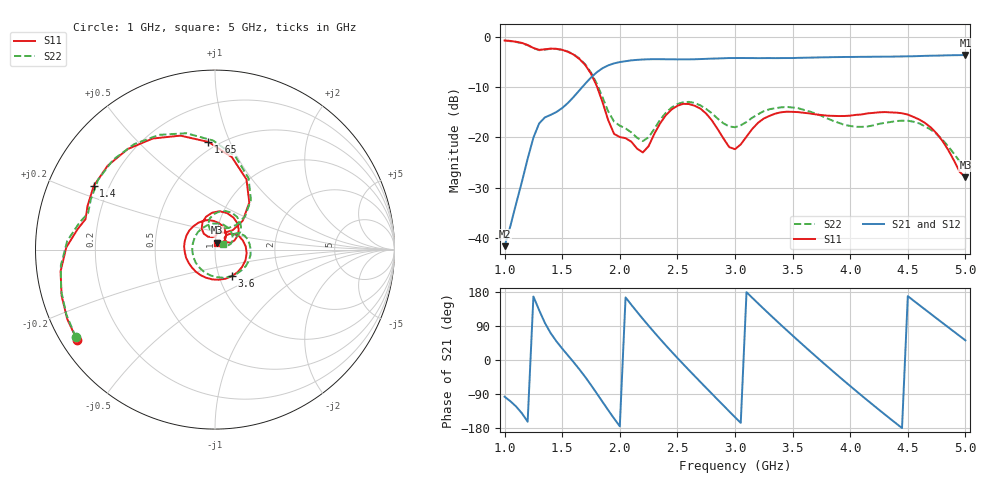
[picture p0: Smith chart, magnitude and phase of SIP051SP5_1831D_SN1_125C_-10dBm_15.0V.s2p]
# GHz  S  dB  R  50
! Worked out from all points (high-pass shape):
!   81 points, 1 GHz to 5 GHz, reference 50 ohm
!   highest |S21| = -3.63 dB at 5 GHz (marker M1); lowest = -41.6 dB at 1 GHz (marker M2)
!   |S21| within 3 dB of the highest: 1.827 GHz to end of sweep
!   lowest |S11| = -27.9 dB at 5 GHz (marker M3), VSWR 1.08, Z = 51.1 + j3.89 ohm
!   |S11| at or under -10 dB: 1.803 GHz to end of sweep
!   |S22| runs from -25.3 to -0.8 dB; largest |S21 - S12| = 0.0015
!   S11 on the Smith chart (normalised r, x): 1 GHz: 0.05, -0.30; 1.4 GHz: 0.14, +0.24; 1.65 GHz: 0.45, +0.84; 3.6 GHz: 1.15, -0.35; 5 GHz: 1.02, +0.08
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1  -0.73 -146.7  -41.65 -97.0  -41.36 -99.5  -0.76 -147.8
1.25  -2.22 171.6  -20.06 167.6  -20.08 167.4  -2.26 168.9
1.4  -2.35 152.3  -15.53 70.8  -15.56 70.8  -2.40 149.2
1.65  -4.42 93.5  -10.63 -25.0  -10.63 -25.0  -4.33 90.9
1.7  -5.62 79.7  -9.33 -44.9  -9.33 -44.9  -5.50 77.7
1.85  -13.02 46.2  -6.25 -110.5  -6.25 -110.5  -12.04 47.8
2.05  -20.16 79.5  -4.86 165.1  -4.85 165.1  -18.21 68.4
2.2  -23.01 101.2  -4.52 108.4  -4.51 108.5  -20.75 86.3
2.35  -17.21 122.6  -4.46 55.4  -4.44 55.4  -16.48 104.4
2.55  -13.34 83.3  -4.49 -10.7  -4.48 -10.7  -13.02 74.1
2.75  -15.29 39.8  -4.38 -73.7  -4.38 -73.7  -14.35 40.8
3  -22.35 41.7  -4.23 -150.9  -4.22 -150.9  -17.99 36.9
3.15  -18.32 46.6  -4.23 164.1  -4.23 164.1  -16.09 35.8
3.35  -15.28 5.7  -4.25 106.4  -4.24 106.3  -14.20 9.4
3.6  -15.12 -57.5  -4.17 37.1  -4.17 37.1  -14.55 -38.3
3.7  -15.43 -82.8  -4.12 10.0  -4.13 10.0  -15.29 -61.0
3.85  -15.73 -119.2  -4.05 -29.8  -4.04 -29.8  -16.70 -99.4
4.05  -15.53 -164.1  -4.00 -81.3  -3.99 -81.4  -17.91 -161.9
4.35  -15.04 132.8  -3.95 -155.6  -3.94 -155.7  -16.95 108.2
4.5  -15.47 102.2  -3.88 168.5  -3.88 168.6  -16.69 71.9
4.7  -18.04 64.2  -3.76 121.5  -3.76 121.6  -18.47 34.0
5  -27.95 71.6  -3.63 51.8  -3.63 51.8  -25.34 38.1
